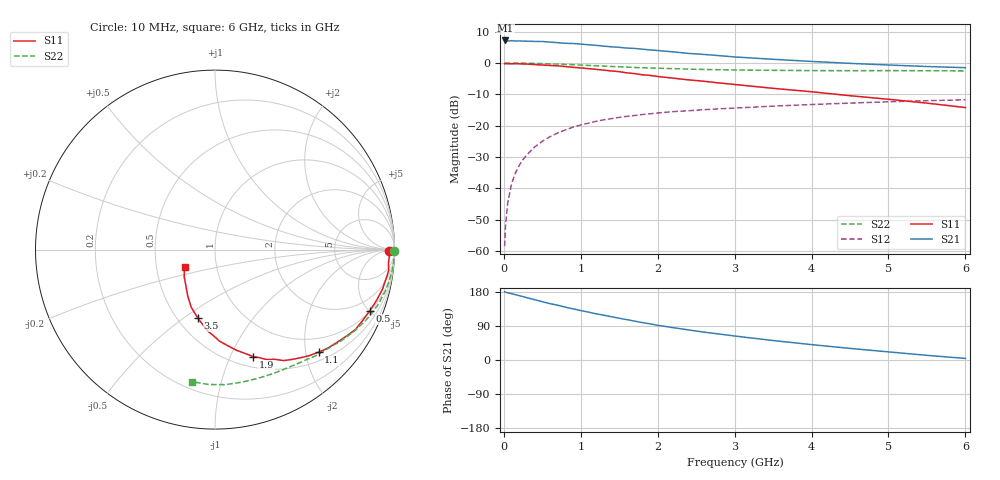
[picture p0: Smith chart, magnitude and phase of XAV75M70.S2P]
! SIEMENS Discrete & RF Semiconductors
! BFY180
! Si NPN RF Bipolar Junction Transistor in MICRO-X
! VCE = 0.75 V  IC = 0.7 mA
! Common Emitter S-Parameters:  May  1997
# GHz  S  MA  R  50
!  f  S11  S21  S12  S22
! GHz  MAG  ANG  MAG  ANG  MAG  ANG  MAG  ANG
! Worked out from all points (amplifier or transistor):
!   36 points, 10 MHz to 6 GHz, reference 50 ohm
!   highest |S21| = 7.2 dB at 20 MHz (marker M1)
!   |S21| within 3 dB of that: start of sweep to 1.896 GHz
!   unconditionally stable (mu >= 1): 3.453 GHz to end of sweep
!   at 250 MHz: K = 0.07, MSG = 18.9 dB, |S12| = -30.8 dB
!   at 1.4 GHz: K = 0.53, MSG = 11.4 dB, |S12| = -17.7 dB
!   at 6 GHz: K = 1.12, MAG = 3.0 dB, |S12| = -11.7 dB
!   S11 on the Smith chart (normalised r, x): 10 MHz: 65, -16; 500 MHz: 1.03, -5.04; 1.1 GHz: 0.67, -2.26; 1.9 GHz: 0.61, -1.22; 3.5 GHz: 0.63, -0.57; 6 GHz: 0.70, -0.14
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0.01  0.9713 -0.4  2.252 179.8  0.0012 87.3  0.9974 -0.3
0.02  0.9762 -0.8  2.285 179.0  0.0024 96.6  0.9999 -0.6
0.05  0.9727 -2.1  2.241 177.7  0.0058 85.7  0.9978 -1.4
0.1  0.9691 -4.5  2.265 175.0  0.0118 88.1  0.9975 -2.8
0.15  0.9746 -6.7  2.239 172.5  0.0176 86.2  0.9977 -4.1
0.2  0.9698 -8.7  2.243 169.7  0.0233 84.3  0.9948 -5.5
0.3  0.9597 -13.1  2.225 164.3  0.0344 80.4  0.9898 -8.1
0.5  0.9275 -21.6  2.199 153.9  0.0564 73.9  0.9779 -13.4
0.6  0.9124 -25.7  2.152 148.6  0.0667 71.0  0.9677 -15.9
0.9  0.8526 -37.5  2.045 135.0  0.0948 62.2  0.9375 -23.1
1.1  0.8123 -44.7  1.951 126.3  0.1098 56.9  0.9135 -27.5
1.2  0.7902 -48.4  1.909 122.0  0.1176 54.4  0.9027 -29.8
1.5  0.7267 -58.3  1.776 110.1  0.1359 47.9  0.8693 -35.5
1.7  0.6764 -64.9  1.705 102.6  0.1452 44.5  0.8472 -39.0
1.9  0.6333 -70.3  1.616 95.5  0.1547 41.0  0.8313 -42.4
2.2  0.5731 -78.0  1.503 85.4  0.1675 36.3  0.8125 -47.2
2.6  0.5112 -87.1  1.368 73.6  0.18 31.5  0.7885 -52.8
2.8  0.48 -91.0  1.308 68.5  0.1857 29.4  0.7799 -55.6
3.5  0.394 -104.0  1.145 51.4  0.2051 22.6  0.7628 -64.9
4.5  0.3006 -120.3  0.986 30.6  0.2291 13.5  0.7536 -78.4
5.5  0.229 -138.5  0.878 12.3  0.2503 4.6  0.7522 -92.6
6  0.1946 -150.7  0.841 4.2  0.2587 0.2  0.7473 -99.7
